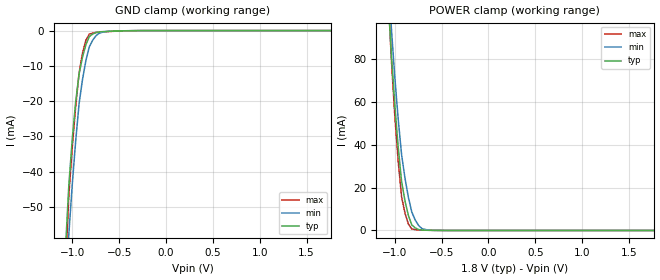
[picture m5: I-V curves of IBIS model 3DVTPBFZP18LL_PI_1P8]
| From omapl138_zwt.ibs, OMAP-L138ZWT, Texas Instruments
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|   Model Cell 3DVTPBFZP18LL_PI_1P8
|IC1833DVTPBFZP18LL_PI_1P8
[Model]   3DVTPBFZP18LL_PI_1P8
Model_type   Input
Polarity   Non-Inverting
Vinl =  0.63
Vinh =  1.17
C_comp   1.254226p   1.200533p   1.264851p
[Model Spec]
Vinl   0.63   0.567   0.693
Vinh   1.17   1.053   1.287
[Temperature Range]   25   125   -40
[Voltage Range]   1.8   1.62   1.98
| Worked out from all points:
|   GND clamp passes 1 mA (typ) near -0.78 V on its own axis
|   POWER clamp passes 1 mA (typ) near -0.77 V on its own axis
[POWER_clamp]
|   voltage   I(typ)   I(min)   I(max)
-1.8V     812.4mA    848.7mA    874.6mA
-1.073V   110mA      121.8mA    111.2mA
-1.036V   81.87mA    94.3mA     79.67mA
-1V       58.6mA     71.62mA    53.64mA
-963.6mV  38.92mA    51.96mA    32.32mA
-927.3mV  22.83mA    35.31mA    15.72mA
-890.9mV  13.72mA    24.34mA    8.029mA
-854.5mV  6.965mA    15.43mA    3.028mA
-818.2mV  2.574mA    8.576mA    711.8uA
-745.5mV  422.4uA    2.295mA    207.6uA
-636.4mV  79.03uA    182.4uA    97.99uA
1.764V    -25.75pA   -519.3nA   -132.1pA
[GND_clamp]
|   voltage   I(typ)   I(min)   I(max)
-1.8V     -593.4mA   -494.6mA   -853.3mA
-1.073V   -62.13mA   -74.14mA   -68.26mA
-1.036V   -43.76mA   -57.65mA   -46.65mA
-1V       -30.75mA   -43.64mA   -33.1mA
-963.6mV  -20.27mA   -31.35mA   -21.56mA
-927.3mV  -12.32mA   -20.76mA   -12.03mA
-890.9mV  -7.558mA   -13.89mA   -6.391mA
-854.5mV  -4.019mA   -8.509mA   -2.715mA
-818.2mV  -1.706mA   -4.609mA   -1.003mA
-745.5mV  -545.1uA   -1.421mA   -528.1uA
-600mV    -195.8uA   -181.2uA   -256.1uA
1.764V    17.31nA    68.32nA    24.84nA
